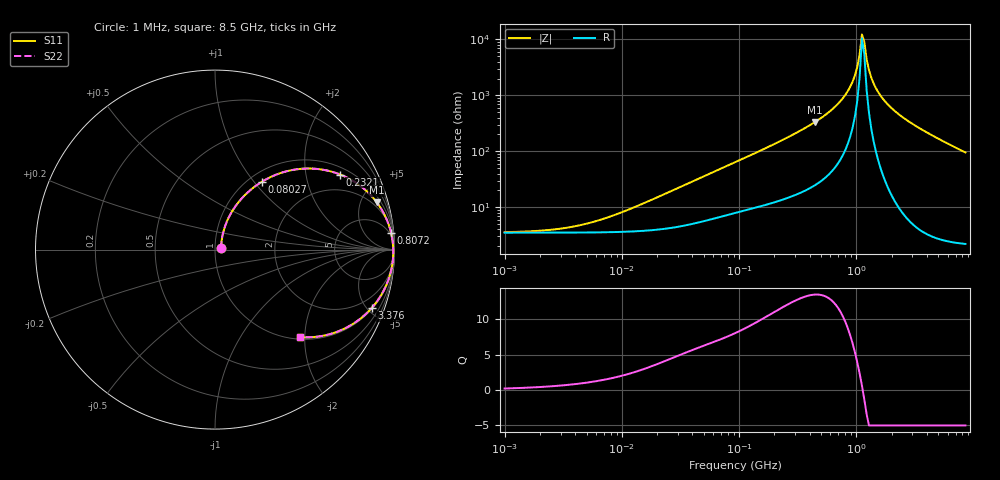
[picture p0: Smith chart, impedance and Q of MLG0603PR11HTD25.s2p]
! S-Parameter Data Generated by TDK Corporation
! Copyright(C) 2025 TDK Corporation.
! All Rights Reserved.
! TDK P/N: MLG0603PR11HTD25 (SMD / SMT Inductor (Coil))
! Property: L=110nH at 300MHz
! Size(LxWxT): 0.6x0.3x0.3mm
! Model Type: s2p (Touchstone File Format Version 1.0)
! Frequency: DC=Yes Start=1MHz Stop=8500MHz 198points Log-sweep
! Model Generated on Feb. 6, 2025
! Terms and conditions regarding TDK Simulation Models:
! 1)This simulation model is being provided solely for informational
!  purposes. Please refer to the specifications of the products in
!  terms of detailed characteristics of such products.
! 2)In no event shall TDK Corporation of any of its subsidiaries be
!  liable for any loss or damage arising, directly or indirectly,
!  from any information contained in this simulation model, including,
!  but not limited to loss or damages arising from any inaccuracies,
!  omissions or errors in connection with such information.
! 3)Any and all copyrights on this simulation model are owned by
!  TDK Corporation.  Duplication or redistribution of this simulation
!  model without prior written permission from TDK Corporation
!  is prohibited.
! 4)This simulation model is subject to any modification or change
!  without any prior notice.
! 5)Neither TDK Corporation nor any of its subsidiaries shall make any
!  warranty, express or implied, including but not limited to the
!  correctness, implied warranties of merchantability and fitness for
!  a particular purpose with respect to this simulation models.
! 6)The use of this simulation model shall be deemed to have consented
!  to the terms and conditions hereof.
! Port Assignments:
!  1 ---@@@--- 2
! Applicable Conditions:
!  Temperature = 25 degC
!  DC Bias Current = 0 A
!  Small Signal Operation
# Hz S MA R 50
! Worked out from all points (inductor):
!   197 points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, 1 MHz to 8.5 GHz, reference 50 ohm
!   read as one part in series: L = 115 nH near 15.95 MHz
!   highest Q = 13.5 at 442.9 MHz (marker M1), where L = 119 nH
!   self-resonance near 1.115 GHz
!   S11 on the Smith chart (normalised r, x): 1 MHz: 1.07, +0.01; 80.27 MHz: 1.15, +1.10; 232.1 MHz: 1.27, +3.14; 807.2 MHz: 3, +20; 3.376 GHz: 1.08, -5.32; 8.5 GHz: 1.04, -1.90
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1000000  0.03455 11.4  0.9661 -0.4  0.9661 -0.4  0.03455 11.4
4587603  0.04691 41.6  0.9654 -1.8  0.9654 -1.8  0.04691 41.6
2.10461e7  0.1496 66.9  0.9513 -8.3  0.9513 -8.3  0.1496 66.9
4.404946e7  0.2876 63.9  0.9109 -16.5  0.9109 -16.5  0.2876 63.9
8.027222e7  0.4607 55.3  0.8293 -27.2  0.8293 -27.2  0.4607 55.3
9.219544e7  0.5074 52.6  0.8011 -30.2  0.8011 -30.2  0.5074 52.6
2.320976e8  0.8135 30.9  0.516 -54.1  0.516 -54.1  0.8135 30.9
4.229561e8  0.9328 17.3  0.2976 -68.5  0.2976 -68.5  0.9328 17.3
4.429384e8  0.9388 16.3  0.2819 -69.4  0.2819 -69.4  0.9388 16.3
6.408078e8  0.9734 9.4  0.1637 -76.0  0.1637 -76.0  0.9734 9.4
8.071757e8  0.9855 5.5  0.09577 -78.6  0.09577 -78.6  0.9855 5.5
9.270694e8  0.99 3.2  0.05657 -78.2  0.05657 -78.2  0.99 3.2
1.016736e9  0.9919 1.7  0.03098 -74.0  0.03098 -74.0  0.9919 1.7
1.064771e9  0.9926 1.0  0.01858 -66.0  0.01858 -66.0  0.9926 1.0
1.115076e9  0.9931 0.2  0.008098 -30.9  0.008098 -30.9  0.9931 0.2
1.167757e9  0.9933 -0.5  0.01096 52.4  0.01096 52.4  0.9933 -0.5
1.222927e9  0.9934 -1.2  0.02261 72.5  0.02261 72.5  0.9934 -1.2
1.34121e9  0.993 -2.7  0.04818 80.3  0.04818 80.3  0.993 -2.7
1.540426e9  0.9909 -5.0  0.08792 81.6  0.08792 81.6  0.9909 -5.0
1.940355e9  0.9829 -9.1  0.1576 79.3  0.1576 79.3  0.9829 -9.1
3.37643e9  0.9312 -20.5  0.3504 68.6  0.3504 68.6  0.9312 -20.5
8.5e9  0.6819 -45.7  0.7158 43.0  0.7158 43.0  0.6819 -45.7
